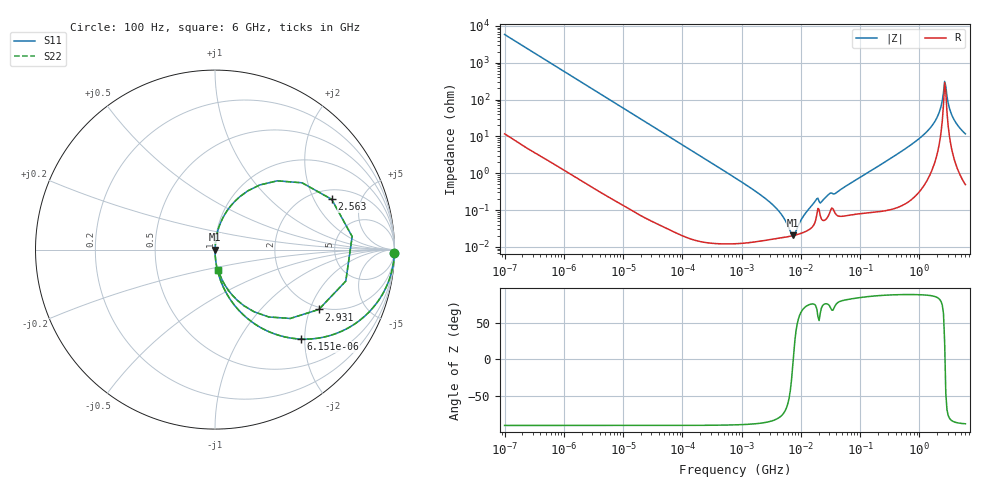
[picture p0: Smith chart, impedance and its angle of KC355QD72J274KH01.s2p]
!Murata Part Number: KC355QD72J274KH01
!These Parameters are Measured in Series Mode Connection
!Data Generated on Mar 13, 2026
!  o--ll--o
!Port1  Port2
!  o------o
!Operation Temp=25[degC], DC Bias Voltage=0[V]
!Freq. Start=100[Hz] Stop=6[GHz] 401[Steps]
# Hz S RI R 50
!Freq.(Hz) S11(Real) S11(Imag) S21(Real) S21(Imag) S12(Real) S12(Imag) S22(Real) S22(Imag)
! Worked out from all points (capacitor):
!   401 points, 100 Hz to 6 GHz, reference 50 ohm
!   read as one part in series: C = 272 nF near 109 Hz
!   lowest |Z| = 20.4 mohm at 7.267 MHz (marker M1)
!   series resonance near 7.452 MHz, so ESL is about 1.7 nH
!   S11 on the Smith chart (normalised r, x): 100 Hz: open; 6.151 kHz: 1.00, -1.91; 2.563 GHz: 2.48, +2.79; 2.931 GHz: 1.92, -2.31; 6 GHz: 1.01, -0.23
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100  0.9997 -0.0171  0.000326 0.0171  0.000326 0.0171  0.9997 -0.0171
600  0.9895 -0.1011  0.0105 0.1011  0.0105 0.1011  0.9895 -0.1011
2008  0.8948 -0.3057  0.1052 0.3057  0.1052 0.3057  0.8948 -0.3057
6151  0.4777 -0.4984  0.5223 0.4984  0.5223 0.4984  0.4777 -0.4984
14402  0.1438 -0.3498  0.8562 0.3498  0.8562 0.3498  0.1438 -0.3498
40335  0.0213 -0.143  0.9787 0.143  0.9787 0.143  0.0213 -0.143
774597  0.000178 -0.00753  0.9998 0.00753  0.9998 0.00753  0.000178 -0.00753
3549919  0.000165 -0.00127  0.9998 0.00127  0.9998 0.00127  0.000165 -0.00127
4856642  0.000178 -0.000688  0.9998 0.000688  0.9998 0.000688  0.000178 -0.000688
7266822  0.000201 -3.88e-05  0.9998 3.88e-05  0.9998 3.88e-05  0.000201 -3.88e-05
1.555665e7  0.000345 0.00132  0.9997 -0.00132  0.9997 -0.00132  0.000345 0.00132
1.779312e7  0.000527 0.00173  0.9995 -0.00173  0.9995 -0.00173  0.000527 0.00173
2.225763e7  0.000575 0.00155  0.9994 -0.00155  0.9994 -0.00155  0.000575 0.00155
3.124326e8  0.00158 0.0239  0.9984 -0.0239  0.9984 -0.0239  0.00158 0.0239
9.569533e8  0.0096 0.0817  0.9904 -0.0817  0.9904 -0.0817  0.0096 0.0817
1.712697e9  0.0566 0.1995  0.9434 -0.1995  0.9434 -0.1995  0.0566 0.1995
2.240541e9  0.2494 0.3601  0.7506 -0.3601  0.7506 -0.3601  0.2494 0.3601
2.562649e9  0.6501 0.2802  0.3499 -0.2802  0.3499 -0.2802  0.6501 0.2802
2.931063e9  0.5782 -0.3337  0.4218 0.3337  0.4218 0.3337  0.5782 -0.3337
3.205649e9  0.2997 -0.3753  0.7003 0.3753  0.7003 0.3753  0.2997 -0.3753
3.666503e9  0.1239 -0.2822  0.8761 0.2822  0.8761 0.2822  0.1239 -0.2822
6e9  0.0181 -0.114  0.9819 0.114  0.9819 0.114  0.0181 -0.114
